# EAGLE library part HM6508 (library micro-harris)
MICROCONTROLLER/MEMORY DEVICE
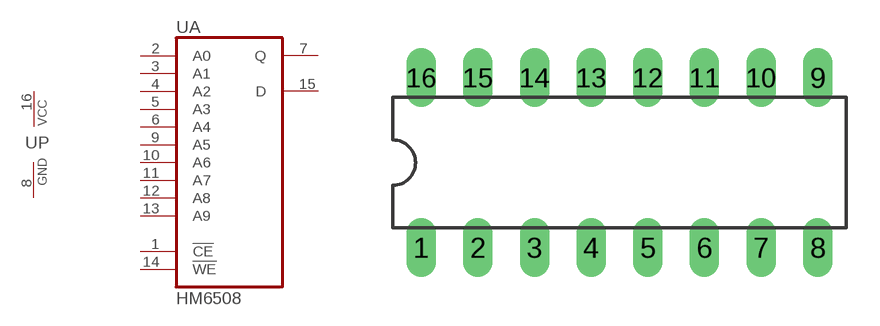
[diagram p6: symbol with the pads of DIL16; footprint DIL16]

Designator prefix U; gates A=HM6508 P=PWRN

## HM6508 (OC_FARNELL: unknown; OC_NEWARK: unknown)  [DIL16]
1  A:!CE  in
2  A:A0  in
3  A:A1  in
4  A:A2  in
5  A:A3  in
6  A:A4  in
7  A:Q  hiz
8  P:GND  pwr
9  A:A5  in
10  A:A6  in
11  A:A7  in
12  A:A8  in
13  A:A9  in
14  A:!WE  in
15  A:D  in
16  P:VCC  pwr

## Footprint DIL16 (pad centres in mm)
Dual In Line Package
drill 0.813 long: 1 -8.89,-3.81; 2 -6.35,-3.81; 3 -3.81,-3.81; 4 -1.27,-3.81; 5 1.27,-3.81; 6 3.81,-3.81; 7 6.35,-3.81; 8 8.89,-3.81; 9 8.89,3.81; 10 6.35,3.81; 11 3.81,3.81; 12 1.27,3.81; 13 -1.27,3.81; 14 -3.81,3.81; 15 -6.35,3.81; 16 -8.89,3.81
